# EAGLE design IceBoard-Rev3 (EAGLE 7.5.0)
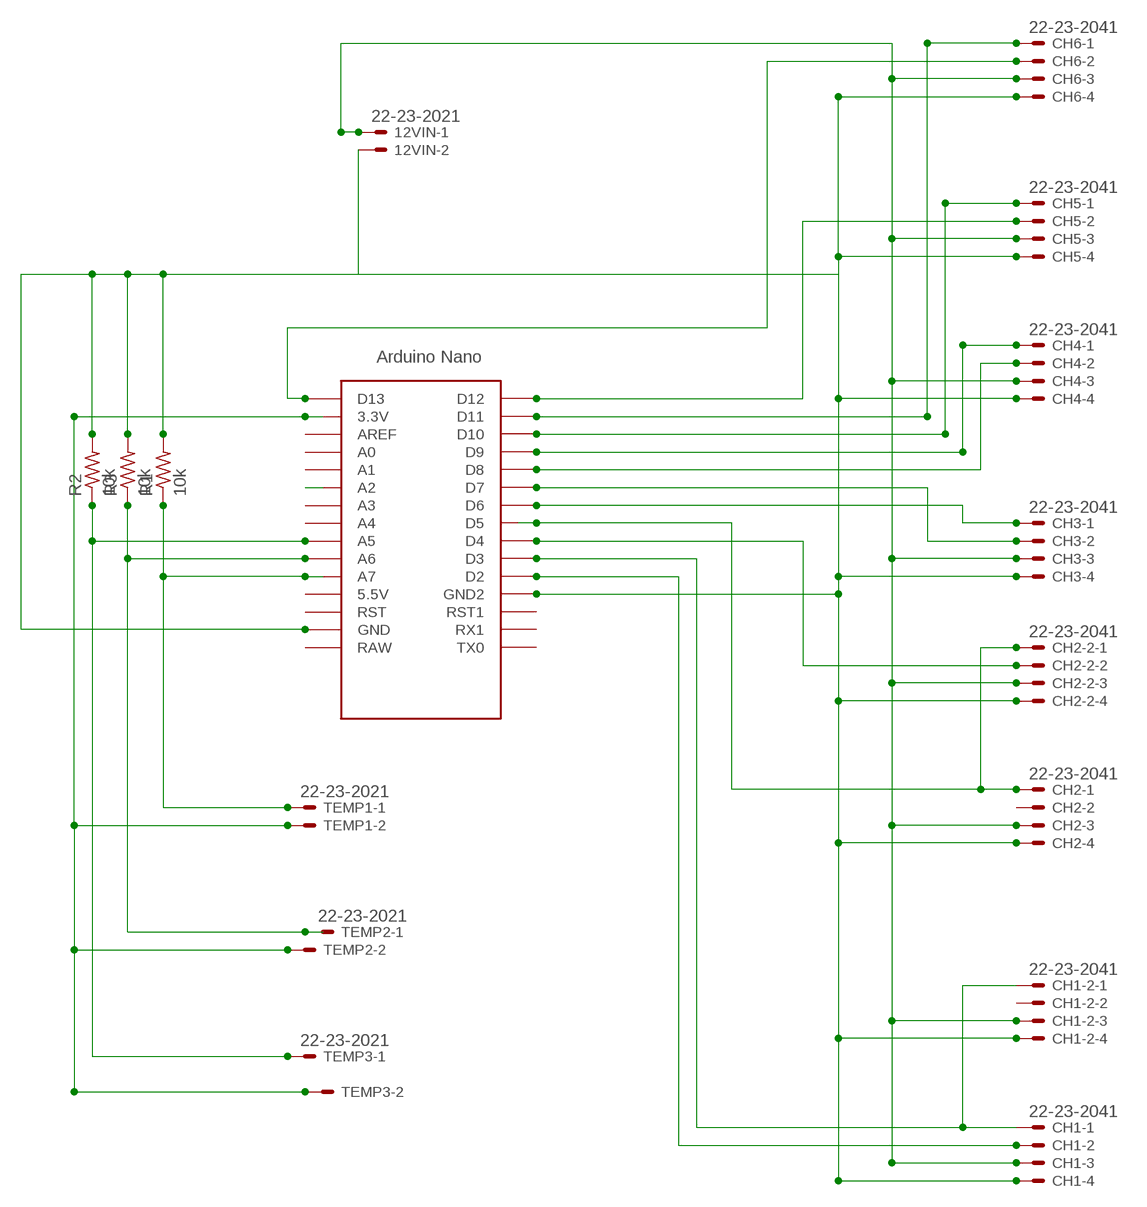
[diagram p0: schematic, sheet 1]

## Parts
12VIN  22-23-2021  [22-23-2021]
CH1  22-23-2041  [22-23-2041]
CH1-2  22-23-2041  [22-23-2041]
CH2  22-23-2041  [22-23-2041]
CH2-2  22-23-2041  [22-23-2041]
CH3  22-23-2041  [22-23-2041]
CH4  22-23-2041  [22-23-2041]
CH5  22-23-2041  [22-23-2041]
CH6  22-23-2041  [22-23-2041]
R1  10k  R-US_R0805  [R0805]
R2  10k  R-US_R0805  [R0805]
R3  10k  R-US_R0805  [R0805]
TEMP1  22-23-2021  [22-23-2021]
TEMP2  22-23-2021  [22-23-2021]
TEMP3  22-23-2021  [22-23-2021]
U$1  NANO  [NANO]

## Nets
10K: TEMP1.2 TEMP2.2 TEMP3.2 U$1.3.3V
GND: 12VIN.2 CH1-2.4 CH1.4 CH2-2.4 CH2.4 CH3.4 CH4.4 CH5.4 CH6.4 R1.2 R2.2 R3.2 U$1.GND U$1.GND1(GND2)
N$1: CH5.1 U$1.D10
N$2: CH6.1 U$1.D11
N$3: CH1-2.1 CH1.1 U$1.D3
N$4: CH2-2.1 CH2.1 U$1.D5
N$5: CH3.1 U$1.D6
N$6: CH4.1 U$1.D9
N$7: R3.1 TEMP2.1 U$1.A6
N$8: 12VIN.1 CH1-2.3 CH1.3 CH2-2.3 CH2.3 CH3.3 CH4.3 CH5.3 CH6.3
N$9: CH6.2 U$1.D13
N$10: CH5.2 U$1.D12
N$11: R1.1 TEMP1.1 U$1.A7
N$12: CH4.2 U$1.D8
N$13: CH3.2 U$1.D7
N$14: CH2-2.2 U$1.D4
N$15: CH1.2 U$1.D2
N$16: U$1.A2
N$18: R2.1 TEMP3.1 U$1.A5
Unconnected: CH1-2.2 CH2.2 U$1.5V(5.5V) U$1.A0 U$1.A1 U$1.A3 U$1.A4 U$1.AREF U$1.ICSP1 U$1.ICSP2 U$1.ICSP3 U$1.ICSP4 U$1.ICSP5 U$1.ICSP6 U$1.RAW U$1.RST U$1.RST1 U$1.RX1 U$1.TX0

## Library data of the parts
12VIN TEMP1-TEMP3 = con-molex:22-23-2021: .100" (2.54mm) Center Header - 2 Pin; MF: MOLEX; MPN: 22-23-2021; OC_FARNELL: 1462926; OC_NEWARK: 25C3832
CH1 CH1-2 CH2 CH2-2 CH3-CH6 = con-molex:22-23-2041: .100" (2.54mm) Center Header - 4 Pin; MF: MOLEX; MPN: 22-23-2041; OC_FARNELL: 1462920; OC_NEWARK: 38C0355
R1-R3 = resistor:R-US_: RESISTOR, American symbol
U$1 = Arduino-clone:NANO: Arduino Nano

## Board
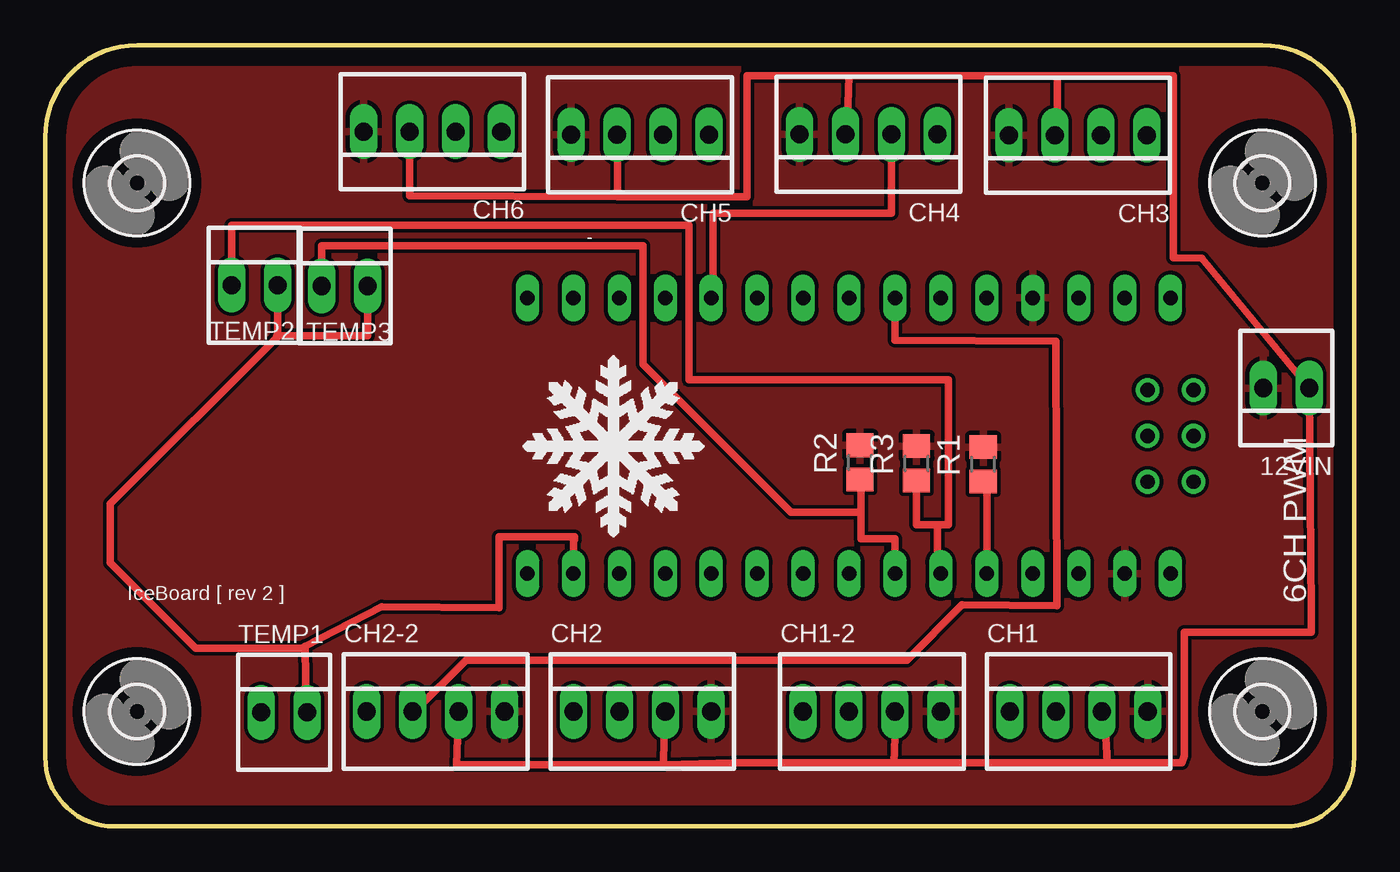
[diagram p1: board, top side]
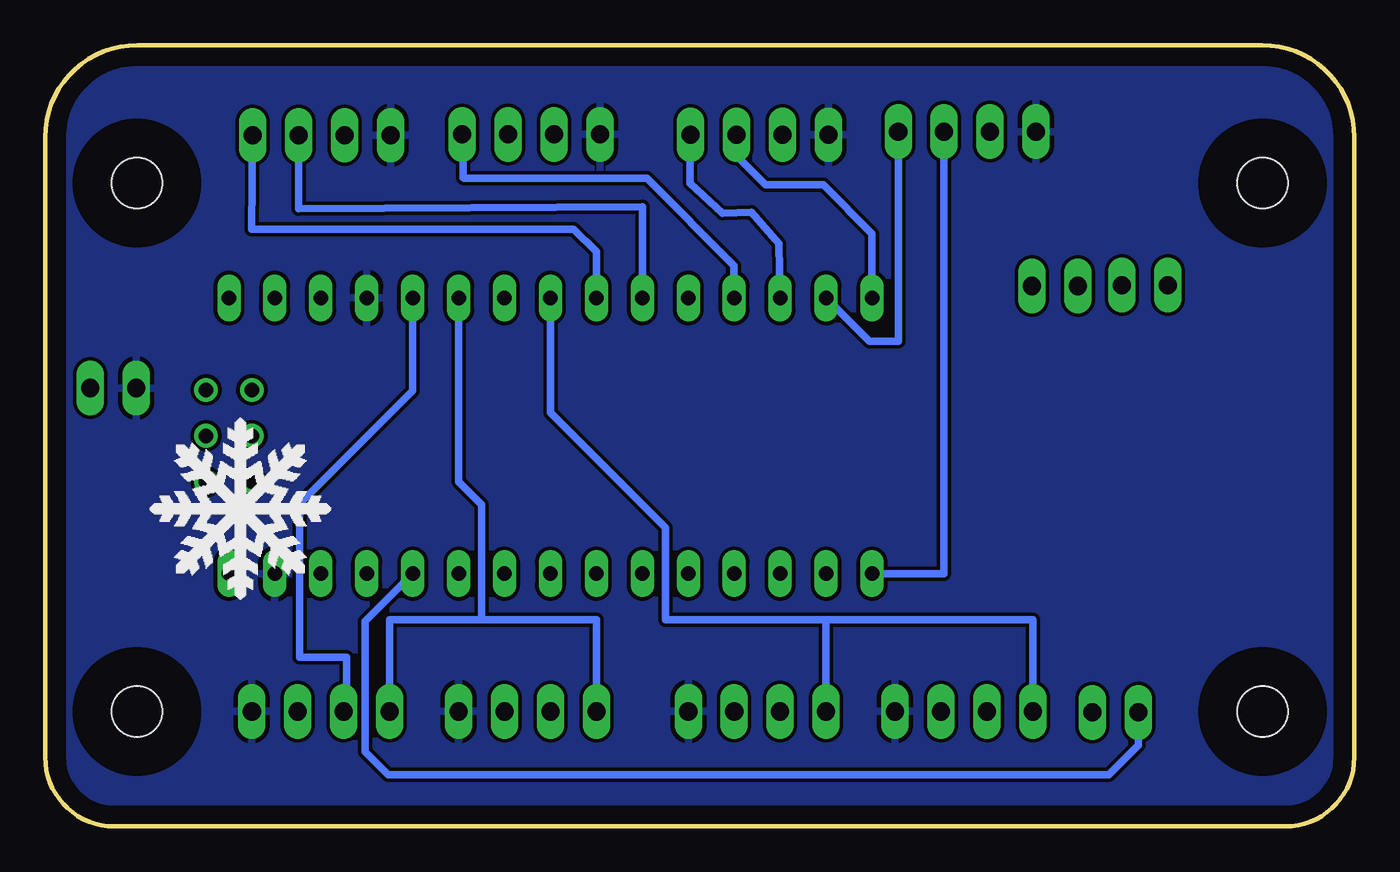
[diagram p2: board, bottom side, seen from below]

Size 72.39 x 43.18 mm. Coordinates in mm from the lower left corner, seen from the top.
Outline: 0,38.1 0,3.81 arc90 3.81,0 68.58,0 arc90 72.39,3.81 72.39,38.1 arc90 67.31,43.18 5.08,43.18 arc90 0,38.1
Copper layers (1*16): Top 0.035mm / dielectric 1.5mm / Bottom 0.035mm
Design rules "default": minimum track width 10mil, minimum drill 24mil, track to track 8mil, track to pad 8mil, pad to pad 8mil, via to via 8mil, smd to smd 8mil, copper to edge 40mil, drill to drill 8mil, minimum pad ring 10mil, minimum via ring 8mil, stop-mask expansion 4mil, vias tented up to drill 0mil, thermal gap 10mil

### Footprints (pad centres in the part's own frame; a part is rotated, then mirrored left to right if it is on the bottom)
22-23-2021 = drill 1 long: 1 -1.27,0; 2 1.27,0
22-23-2041 = drill 1 long: 1 -3.81,0; 2 -1.27,0; 3 1.27,0; 4 3.81,0
R0805 = smd 1.3 x 1.5: 1 -0.95,0; 2 0.95,0
NANO = drill 0.8 long: 3.3V -10.16,24.13; 5V -10.16,-1.27; A0 -10.16,19.05; A1 -10.16,16.51; A2 -10.16,13.97; A3 -10.16,11.43; A4 -10.16,8.89; A5 -10.16,6.35; A6 -10.16,3.81; A7 -10.16,1.27; AREF -10.16,21.59; D2 5.08,1.27; D3 5.08,3.81; D4 5.08,6.35; D5 5.08,8.89; D6 5.08,11.43; D7 5.08,13.97; D8 5.08,16.51; D9 5.08,19.05; D10 5.08,21.59; D11 5.08,24.13; D12 5.08,26.67; D13 -10.16,26.67; GND -10.16,-6.35; GND1 5.08,-1.27; RAW -10.16,-8.89; RST -10.16,-3.81; RST1 5.08,-3.81; RX1 5.08,-6.35; TX0 5.08,-8.89 | drill 0.8: ICSP1 -5.08,-10.16; ICSP2 -5.08,-7.62; ICSP3 -2.54,-10.16; ICSP4 -2.54,-7.62; ICSP5 0,-10.16; ICSP6 0,-7.62
2,8 = hole 2.8: 0,0

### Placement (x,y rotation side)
12VIN  68.63,24.23 180 top
CH1  57.15,6.35 0 top
CH1-2  45.72,6.35 0 top
CH2  33.02,6.35 0 top
CH2-2  21.59,6.35 0 top
CH3  57.1,38.2 180 top
CH4  45.52,38.25 180 top
CH5  32.89,38.23 180 top
CH6  21.41,38.4 180 top
R1  51.87,20.02 90 top
R2  45.06,20.12 90 top
R3  48.18,20.07 90 top
TEMP1  13.21,6.3 0 top
TEMP2  11.58,29.92 0 top
TEMP3  16.56,29.87 0 top
U$1  53.34,24.13 90 top
U$2  [2,8]  5.08,35.56 0 top
U$3  [2,8]  5.08,6.35 0 top
U$4  [2,8]  67.31,6.35 0 top
U$5  [2,8]  67.31,35.56 0 top

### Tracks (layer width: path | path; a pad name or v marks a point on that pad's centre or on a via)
10K
  Top 0.406: TEMP1.2 14.43,6.35 14.38,9.96 | 14.38,9.96 18.59,12.14 25.09,12.09 25.09,16 29.26,16 29.26,15.85 29.21,15.85 U$1.3.3V | 12.9,27.13 12.8,27.13 12.85,27.18 TEMP2.2 | TEMP3.2 17.83,27.13 12.9,27.13 | 12.9,27.13 3.61,17.83 3.61,14.58 8.33,9.86 14.38,9.86 14.38,9.96
GND
  Top 0.254: 59.64,13.92 U$1.GND
  pour Bottom: 0.05,38.02 arc-90 5.16,43.13 67.21,43.13 arc-90 72.42,37.92 72.42,3.91 arc-90 68.45,-0.05 3.71,-0.05 arc-90 0,3.66 0.05,32.41
  pour Top: -0.05,37.34 arc-90 5.79,43.18 7.37,43.18 arc90 7.42,43.13 67.41,43.13 arc-90 72.39,38.15 72.39,3.15 arc-90 69.19,-0.05 3.66,-0.05 arc-90 0.05,3.56
N$1
  Bottom 0.406: CH5.1 36.73,38.2 36.73,35.56 34.95,33.88 33.32,33.93 31.8,32.21 U$1.D10
N$2
  Bottom 0.406: CH6.1 25.2,31.75 25.2,26.82 26.82,26.82 U$1.D11
N$3
  Bottom 0.406: CH1-2.1 41.91,11.43 48.26,11.43 | CH1.1 53.34,11.43 48.26,11.43 | U$1.D3 49.53,19.05 48.26,17.78 48.26,11.43
N$4
  Bottom 0.406: U$1.D5 44.45,22.86 38.1,16.51 38.1,11.43 29.21,11.43 | 29.21,11.43 17.78,11.43 CH2-2.1 | CH2.1 29.21,11.43
N$5
  Bottom 0.406: U$1.D6 41.91,31.75 43.18,33.02 60.96,33.02 CH3.1
N$6
  Bottom 0.406: 49.53,38.1 CH4.1 49.28,38.2 49.28,35.87 49.22,35.81 39.12,35.81 34.29,30.99 U$1.D9
N$7
  Top 0.406: TEMP2.1 10.31,33.22 35.61,33.22 35.61,24.69 49.94,24.69 49.94,16.66 49.33,16.66 | 49.33,16.66 49.33,13.97 U$1.A6 | R3.1 48.18,16.66 49.33,16.66
N$8
  Top 0.406: 58.72,3.51 62.84,3.51 62.99,3.91 62.99,10.72 70,10.72 70,11.84 12VIN.1 63.96,31.39 62.38,31.45 62.38,41.5 55.98,41.5 | 58.72,3.51 46.94,3.51 | 46.94,3.51 38.05,3.51 34.19,3.4 | 34.19,3.4 22.76,3.4 CH2-2.3 | CH2.3 34.24,6.35 34.19,3.4 | CH1.3 58.57,6.35 58.72,3.51 | CH1-2.3 47.04,6.35 46.94,3.51 | 55.98,41.5 44.45,41.5 | 44.45,41.5 38.81,41.5 38.81,34.8 31.65,34.8 | 31.65,34.8 20.14,34.85 CH6.3 | CH4.3 44.35,38.25 44.45,41.5 | CH3.3 55.98,38.2 55.98,41.5 | CH5.3 31.65,38.23 31.65,34.8
N$9
  Bottom 0.406: U$1.D13 22.68,13.97 CH6.2
N$10
  Bottom 0.406: 26.72,29.26 U$1.D12 26.67,32.77 29.36,35.46 32.56,35.46 34.16,37.06 CH5.2
N$11
  Top 0.406: 51.99,14.05 U$1.A7 52.07,18.86 R1.1
  Bottom 0.406: TEMP1.1 11.94,4.47 13.56,2.85 53.44,2.85 54.71,4.12 54.71,11.33 U$1.A7
N$12
  Top 0.406: CH4.2 46.79,33.88 36.93,33.88 36.93,29.21 U$1.D8
N$13
  Bottom 0.406: CH3.2 58.37,34.14 39.37,34.24 U$1.D7
N$14
  Top 0.406: CH2-2.2 20.42,6.35 23.27,9.2 47.65,9.2 50.7,12.24 55.93,12.19 55.88,26.82 46.99,26.87 U$1.D4
N$15
  Bottom 0.406: U$1.D2 52.07,24.08 58.32,17.83 58.32,9.35 55.73,9.35 55.73,6.5 CH1.2
N$18
  Top 0.406: U$1.A5 46.99,15.9 45.11,15.9 45.11,17.22 | 45.11,17.22 45.11,19.17 R2.1 | TEMP3.1 15.29,32.11 33.07,32.11 33.07,25.55 41.25,17.37 44.96,17.37 45.11,17.22

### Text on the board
tPlace: IceBoard [ rev 2 ] | 6CH PWM
bPlace: /Users/tink3rbot/Desktop/snowflake.bmp
bStop: [tink3r]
